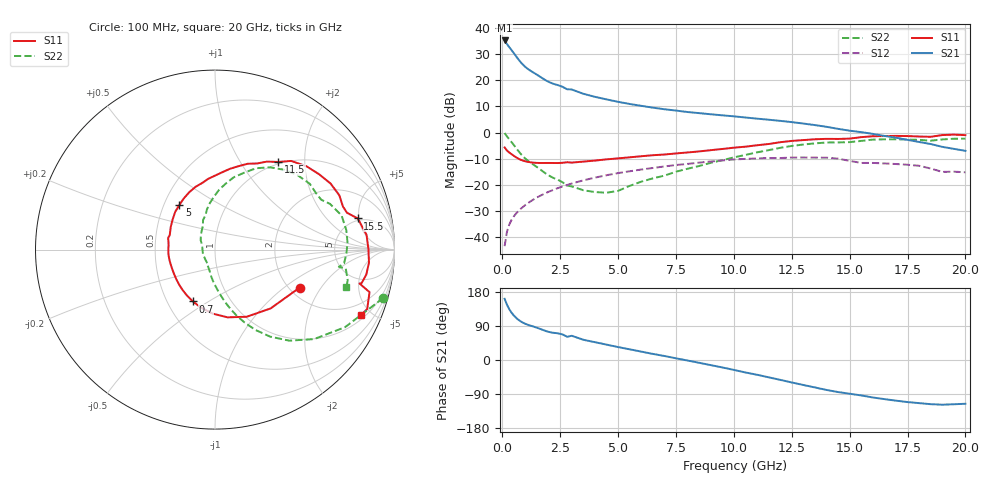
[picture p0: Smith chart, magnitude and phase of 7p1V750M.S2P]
! Infineon Technologies  Discrete & RF Semiconductors
! bfp620
! VCE =  1.7 V,  IC =  50 mA
! Common Emitter S-Parameters:  Sep 2002
# GHz  S  MA  R  50
!  f  S11  S21  S12  S22
! GHz  MAG  ANG  MAG  ANG  MAG  ANG  MAG  ANG
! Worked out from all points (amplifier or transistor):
!   59 points, 100 MHz to 20 GHz, reference 50 ohm
!   highest |S21| = 35.3 dB at 100 MHz (marker M1)
!   |S21| within 3 dB of that: start of sweep to 339.3 MHz
!   unconditionally stable (mu >= 1): 2.672 GHz to 2.972 GHz; 3.046 GHz to 9.822 GHz; 17.18 GHz to end of sweep
!   at 1 GHz: K = 0.85, MSG = 26.5 dB, |S12| = -27.8 dB
!   at 5.5 GHz: K = 1.04, MAG = 11.7 dB, |S12| = -14.9 dB
!   at 20 GHz: K = 1.28, MAG = 0.9 dB, |S12| = -15.3 dB
!   S11 on the Smith chart (normalised r, x): 100 MHz: 2.27, -1.31; 700 MHz: 0.67, -0.43; 5 GHz: 0.60, +0.33; 11.5 GHz: 0.97, +1.48; 15.5 GHz: 4.69, +4.82; 20 GHz: 1.22, -4.32
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0.1  0.5174 -24.1  58.32 161.5  0.0066 77.6  0.9748 -16.1
0.2  0.4511 -46.6  49.82 146.1  0.0124 72.9  0.8439 -30.8
0.3  0.4137 -64.7  43.52 134.1  0.0171 70.0  0.7438 -42.1
0.4  0.3839 -79.5  38.06 124.7  0.0211 67.9  0.6548 -50.8
0.5  0.3569 -92.1  33.15 117.2  0.0247 66.4  0.5734 -57.7
0.6  0.3333 -103.3  28.82 111.1  0.0281 65.3  0.5008 -63.3
0.7  0.3141 -113.1  25.16 105.9  0.0313 64.6  0.4387 -67.9
0.9  0.2882 -129.0  19.85 98.2  0.0376 63.7  0.3467 -75.0
1.1  0.2736 -140.5  16.62 93.0  0.044 63.1  0.2889 -79.8
1.8  0.2602 -168.6  10.53 78.3  0.0664 59.5  0.1729 -94.0
2  0.2606 -175.1  9.365 74.2  0.0729 58.1  0.1503 -98.2
2.8  0.2692 166.0  6.762 61.4  0.0986 51.8  0.0958 -116.1
3  0.2646 162.4  6.677 63.9  0.105 50.0  0.0924 -115.0
3.5  0.2768 153.0  5.531 53.4  0.1209 45.4  0.078 -132.4
5  0.3188 128.5  3.882 34.1  0.1663 31.0  0.0759 160.9
7  0.3783 100.7  2.796 10.6  0.2232 11.6  0.1487 117.0
10.5  0.535 63.8  1.94 -32.9  0.3119 -28.1  0.3716 80.9
11.5  0.6014 54.3  1.76 -45.7  0.3247 -40.5  0.4585 69.2
13.5  0.7415 29.8  1.388 -72.4  0.3298 -64.6  0.6191 42.2
15.5  0.8142 12.3  1.017 -93.5  0.261 -86.8  0.6895 21.7
17  0.861 -4.8  0.794 -107.3  0.2484 -96.4  0.7392 3.0
20  0.8908 -24.3  0.445 -115.5  0.1726 -106.2  0.7611 -15.8
